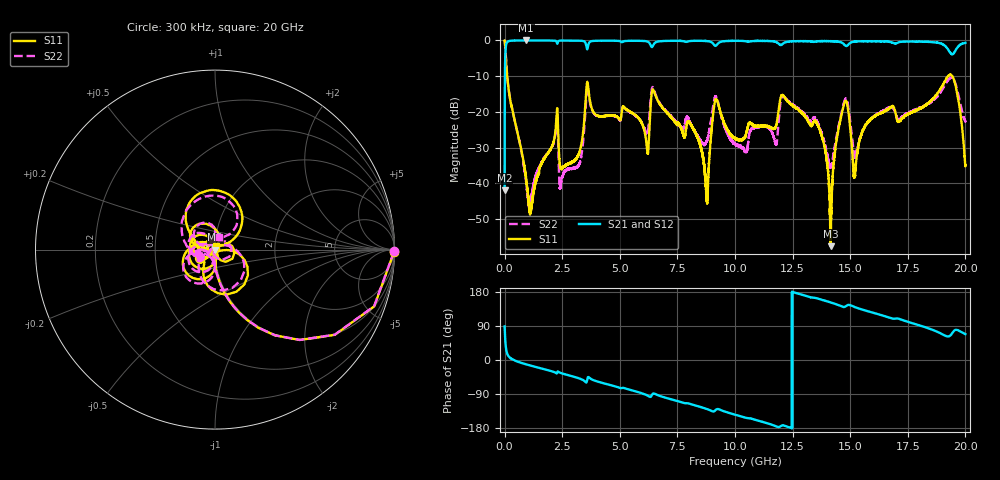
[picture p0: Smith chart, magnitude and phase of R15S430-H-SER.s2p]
!{R15S430}
!Johanson Technology Inc.
!www.johansontechnology.com
!Test Board Conditions:
!Substrate Type  RO4350B
!Substrate Thickness  20 mil
!Substrate Dk  3.66
!TL Type: GCPW
!TL Trace Width  34 mil
!TL Gap  10 mil
!Electrode orientation  Horizontal
!DUT TOPOLOGY	SERIES
!Mounting Pad LxW  26x52 mil
! Created Sat Feb  6 14:28:34 2021
# hz S ma R 50
! 2 Port Network Data from SP1.SP block
! freq  magS11  angS11  magS21  angS21  magS12  angS12  magS22  angS22
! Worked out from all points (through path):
!   20001 points, 300 kHz to 20 GHz, reference 50 ohm
!   highest |S21| = 0.00 dB at 936.3 MHz (marker M1); lowest = -42.0 dB at 300 kHz (marker M2)
!   group delay of S21, straight-line fit = 41.8 ps
!   lowest |S11| = -57.6 dB at 14.15 GHz (marker M3), VSWR 1.00, Z = 50.1 - j0.0782 ohm
!   |S11| at or under -10 dB: 111.6 MHz to 19.24 GHz (19.13 GHz wide, 198 % of centre); 19.43 GHz to end of sweep
!   |S22| runs from -47.0 to 0.0 dB; largest |S21 - S12| = 0.013
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300000  0.9982 -0.6  0.007971 88.6  0.007918 89.2  0.9977 -0.6
1.253e8  0.2842 -75.1  0.9576 14.8  0.9575 14.8  0.2851 -74.9
9.363e8  0.01142 -85.9  0.9997 -11.4  0.9981 -11.4  0.01062 -121.8
1.1433e9  0.004524 1.4  0.9989 -15.0  0.999 -15.0  0.00567 138.8
2.2213e9  0.06028 32.7  0.9846 -33.9  0.9847 -33.9  0.05554 55.4
2.4573e9  0.01607 -24.8  0.9959 -34.6  0.9955 -34.7  0.01062 134.7
3.3343e9  0.03556 -8.0  0.9899 -50.8  0.9896 -50.8  0.02475 62.2
3.6163e9  0.2408 -87.5  0.823 -45.1  0.8229 -45.0  0.2181 -93.6
6.1773e9  0.03156 -163.6  0.9693 -93.0  0.9708 -93.0  0.04945 -129.9
6.6673e9  0.1401 176.5  0.9679 -93.1  0.9689 -93.1  0.1431 -169.1
8.7593e9  0.006281 57.0  0.9806 -129.0  0.9818 -128.9  0.03905 -120.6
9.1673e9  0.1504 -150.9  0.8418 -131.5  0.8432 -131.5  0.1647 -146.9
1.00003e10  0.0427 155.3  0.9873 -144.3  0.988 -144.3  0.03514 116.1
1.17603e10  0.06116 154.7  0.9588 -174.4  0.9558 -174.4  0.03519 111.5
1.20693e10  0.1715 128.3  0.896 -172.6  0.8941 -172.6  0.1655 123.6
1.33343e10  0.06431 88.0  0.9606 165.0  0.9594 164.9  0.07359 103.3
1.41503e10  0.001316 -36.4  0.978 151.9  0.9779 151.9  0.01661 151.8
1.47613e10  0.1362 -179.1  0.8625 140.2  0.8638 140.1  0.1456 175.4
1.51953e10  0.01238 -177.9  0.9661 139.6  0.9618 139.9  0.0238 156.9
1.66673e10  0.1092 -163.9  0.9619 112.3  0.9525 112.4  0.1146 -156.9
1.93783e10  0.3297 87.3  0.6535 66.8  0.6569 67.2  0.3011 99.1
2e10  0.01809 78.3  0.9249 68.3  0.9225 68.2  0.07382 71.5
